// TwinCAT 3 PLC project OOP2
// ProgramVersion: 3.1.4020.2
// libraries:
//   Tc2_Standard, * (Beckhoff Automation GmbH)
//   Tc2_System, * (Beckhoff Automation GmbH)
//   Tc3_Module, * (Beckhoff Automation GmbH)
// project tree:
//   / PlcTask.TcTTO
//   POUs/ FB_Count.TcPOU, FB_CountEX.TcPOU, I_Count.TcIO, MAIN.TcPOU

CONFIGURATION OOP2
    RESOURCE PLC ON TwinCAT3
        TASK PlcTask(INTERVAL := T#10ms, PRIORITY := 20);
        PROGRAM MAIN WITH PlcTask : MAIN;
    END_RESOURCE
END_CONFIGURATION

// ---- POUs/I_Count.TcIO
INTERFACE I_Count

METHOD M_Count : INT
VAR_INPUT
	bEnable: BOOL;
END_VAR
VAR_OUTPUT
	i_Wert, k_Wert: INT;	
END_VAR
END_METHOD

PROPERTY P_Max_i : INT
GET
END_GET
SET
END_SET
END_PROPERTY

PROPERTY P_Max_k : INT
GET
END_GET
SET
END_SET
END_PROPERTY

END_INTERFACE

// ---- POUs/MAIN.TcPOU
PROGRAM MAIN
VAR
	count1: FB_Count; 
	count2: FB_CountEX; 
	icount: I_Count;
	i,k :INT;
	Startcount:BOOL;
	check: BOOL;
	max_i: INT;
	max_k: INT;
	change: BOOL:=TRUE;
END_VAR

IF change THEN
	icount:=count1;
ELSE
	icount:=count2;
	check:=count2.M_Check(bCheckValue:=Startcount );
END_IF
				
icount.M_Count( bEnable:=Startcount ,
	            i_Wert=>i,
				k_Wert=>k );

icount.P_Max_i:=1000;
max_i:=icount.P_Max_i;

icount.P_Max_k:=2000;
max_k:=icount.P_Max_k;

END_PROGRAM

// ---- POUs/FB_Count.TcPOU
FUNCTION_BLOCK FB_Count IMPLEMENTS I_Count
VAR
	i,k: INT;
	max_i:INT:=755;
	max_k: INT:=2265;
END_VAR

{warning 'add method implementation'}
METHOD M_Count : INT
VAR_INPUT
	bEnable	: BOOL;
END_VAR
VAR_OUTPUT
	i_Wert	: INT;
	k_Wert	: INT;
END_VAR
IF bEnable THEN
	i:=i+1;
	IF i>=max_i THEN
		i:=0;
	END_IF
	k:=k+1;
	IF k>=max_k THEN
		k:=0;
	END_IF
	i_Wert:=i;
	k_Wert:=k;
END_IF
END_METHOD

{warning 'add property implementation'}
PROPERTY P_Max_i : INT
GET
P_Max_i:=max_i;
END_GET
SET
max_i:=P_Max_i;
END_SET
END_PROPERTY

{warning 'add property implementation'}
PROPERTY P_Max_k : INT
GET
P_Max_k:=max_k;
END_GET
SET
max_k:=P_Max_k;
END_SET
END_PROPERTY

END_FUNCTION_BLOCK

// ---- POUs/FB_CountEX.TcPOU
FUNCTION_BLOCK FB_CountEX EXTENDS FB_Count
VAR_INPUT
END_VAR
VAR_OUTPUT
END_VAR
VAR
END_VAR

METHOD M_Check : BOOL
VAR_INPUT
	bCheckValue: BOOL;
END_VAR
IF bCheckValue THEN
	IF i=k THEN
		M_Check:=TRUE;
	ELSE
		M_Check:=FALSE;
	END_IF  
END_IF
END_METHOD

END_FUNCTION_BLOCK
